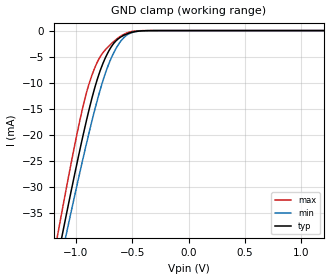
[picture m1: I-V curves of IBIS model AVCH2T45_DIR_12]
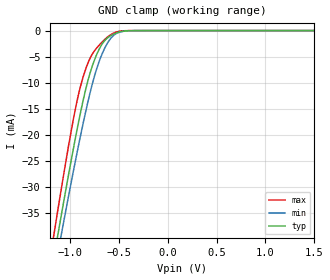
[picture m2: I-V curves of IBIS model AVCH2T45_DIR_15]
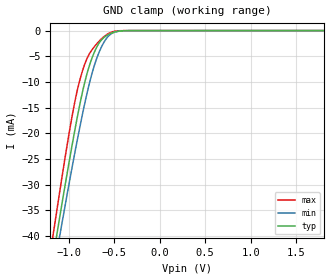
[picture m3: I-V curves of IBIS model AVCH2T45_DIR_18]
| TEXAS INSTRUMENTS INCORPORATED
| Standard Linear and Logic Group
| IBIS Model of SN74AVCH2T45
| DUAL-BIT DUAL-SUPPLY BUS TRANSCEIVER WITH CONFIGURABLE VOLTAGE
| TRANSLATION AND 3-STATE OUTPUTS
| This file contains package information for the following:
|  SOT 8-pin (DCU) package as [Component] AVCH2T45_DCU
|  SOT 8-pin (DCT) package as [Component] AVCH2T45_DCT
|  NanoFree WCSP 8-pin (YZP) package as [Component] AVCH2T45_YZP
| This device can be powered at the following Vccs:
|  1.2 volt Vcc
|  1.5 volt Vcc
|  1.8 volt Vcc
|  2.5 volt Vcc
|  3.3 volt Vcc
| This file provides unique models under the [Model Selector] for each Vcc.
| For operation at a specific Vcc, select the appropriate model after each
| [Model Selector] keyword.
[IBIS Ver]   3.2
[Comment char]  |_char
[File Name]   sn74avch2t45.ibs
[File Rev]   1.2 | x_die
[Date]   December 7, 2005
[Source]   Data created from TI-SPICE simulations at TI-SLL.
[Notes]   The following is an IBIS list for the AVCH2T45.
   Please contact sllibis@ti.com with questions and
   comments concerning SLL IBIS models.
   - FILE REV HISTORY
   - 1.1 Release of IBIS File on 04/29/04
   - 1.2 YZP package added on 12/07/05
   - Power clamp data deleted as there is no power-clamp diode.
   - Due to the fact that the Device is 4.6-V Input/Output
   tolarent, the I/O models has some Non-Monotonic Warnings.
   - Non-monotonic data in ground-clamp due to bus-hold
[Disclaimer] Property of Texas Instruments Incorporated.  Unauthorized
   reproduction and/or distribution is strictly prohibited.
   This product is protected under copyright law.
   Created  2004, (C) Copyright  2004, Texas Instruments
   Incorporated, All Rights Reserved
   UNLESS THERE IS A SIGNED, WRITTEN AGREEMENT TO THE
   CONTRARY, TEXAS INSTRUMENTS (TI) IS PROVIDING THE IBIS
   MODELS  AND WITHOUT ANY WARRANTY, EXPRESSED OR
   IMPLIED.  TI assumes no liability for:
   1) the accuracy of the IBIS models provided to your
   company;
   2) the proper functioning of these IBIS Models in your
   design or for any resulting applications; or
   3) infringement of patents, copyrights or intellectual
   property rights resulting from your use of these IBIS
   models.
   TI provides IBIS Models as a service to our customers.
   You and your company shall not distribute, sell or give
   these models to anyone else without prior written
   permission from TI.
   TI reserves the right to make changes to our products or
   to discontinue any semiconductor product or service
   without notice, and advises our customers to obtain the
   latest version of relevant information to verify, before
   placing orders, that the information being relied on is
   current.
   Please be aware that your receipt and use of the IBIS
   information provided shall serve as acceptance of these
   terms and conditions.  If you do not accept these terms,
   you should return or destroy the IBIS models and any
   other accompanying information immediately.
| Component AVCH2T45_DCU 8-pin SOT
[Component]   AVCH2T45_DCU
[Manufacturer]   Texas Instruments, Inc.
[Package]
|   typ   min   max
R_pkg   2.600e-02   2.300e-02   3.800e-02
L_pkg   1.394e-09   1.066e-09   2.046e-09
C_pkg   2.590e-13   2.150e-13   3.720e-13
[Pin]   signal_name   model_name   R_pin   L_pin   C_pin
1   VCCA   POWER   2.400e-02   1.520e-09   2.710e-13
2   A1   AVCH2T45_IOA   2.300e-02   1.112e-09   2.180e-13
3   A2   AVCH2T45_IOA   2.300e-02   1.070e-09   2.170e-13
4   GND   GND   2.700e-02   2.046e-09   3.720e-13
5   DIR   AVCH2T45_DIR   2.700e-02   1.542e-09   2.730e-13
6   B2   AVCH2T45_IOB   2.300e-02   1.100e-09   2.240e-13
7   B1   AVCH2T45_IOB   2.300e-02   1.066e-09   2.150e-13
8   VCCB   POWER   3.800e-02   1.696e-09   2.800e-13
| Component AVCH2T45_DCT 8-pin SOT
[Component]   AVCH2T45_DCT
[Manufacturer]   Texas Instruments, Inc.
[Package]
|   typ   min   max
R_pkg   2.900e-02   2.800e-02   3.100e-02
L_pkg   1.796e-09   1.666e-09   1.924e-09
C_pkg   2.310e-13   2.210e-13   2.420e-13
[Pin]   signal_name   model_name   R_pin   L_pin   C_pin
1   VCCA   POWER   3.100e-02   1.894e-09   2.230e-13
2   A1   AVCH2T45_IOA   2.800e-02   1.697e-09   2.370e-13
3   A2   AVCH2T45_IOA   3.000e-02   1.722e-09   2.390e-13
4   GND   GND   3.000e-02   1.861e-09   2.210e-13
5   DIR   AVCH2T45_DIR   2.800e-02   1.924e-09   2.280e-13
6   B2   AVCH2T45_IOB   2.900e-02   1.736e-09   2.420e-13
7   B1   AVCH2T45_IOB   2.800e-02   1.666e-09   2.360e-13
8   VCCB   POWER   3.000e-02   1.871e-09   2.220e-13
| Component AVCH2T45_YZP 8-pin NanoFree WCSP
[Component]   AVCH2T45_YZP
[Manufacturer]   Texas Instruments, Inc.
[Package]
|   typ   min   max
R_pkg   0.001   0.001   0.001
L_pkg   0.021nH   0.021nH   0.021nH
C_pkg   0.043pF   0.042pF   0.044pF
[Pin]   signal_name   model_name   R_pin   L_pin   C_pin
1   VCCA   POWER   0.046   2.861nH   0.321pF
2   A1   AVCH2T45_IOA   0.037   2.437nH   0.286pF
3   A2   AVCH2T45_IOA   0.034   2.419nH   0.286pF
4   GND   GND   0.043   2.784nH   0.321pF
5   DIR   AVCH2T45_DIR   0.043   2.784nH   0.321pF
6   B2   AVCH2T45_IOB   0.035   2.420nH   0.286pF
7   B1   AVCH2T45_IOB   0.037   2.437nH   0.286pF
8   VCCB   POWER   0.046   2.860nH   0.321pF
| Model AVCH2T45_DIR
[Model Selector]   AVCH2T45_DIR
AVCH2T45_DIR_12   1.2 volt Vcc
AVCH2T45_DIR_15   1.5 volt Vcc
AVCH2T45_DIR_18   1.8 volt Vcc
AVCH2T45_DIR_25   2.5 volt Vcc
AVCH2T45_DIR_33   3.3 volt Vcc
| Model AVCH2T45_IOA
[Model Selector]   AVCH2T45_IOA
AVCH2T45_IOA_12   1.2 volt Vcc
AVCH2T45_IOA_15   1.5 volt Vcc
AVCH2T45_IOA_18   1.8 volt Vcc
AVCH2T45_IOA_25   2.5 volt Vcc
AVCH2T45_IOA_33   3.3 volt Vcc
| Model AVCH2T45_IOB
[Model Selector]   AVCH2T45_IOB
AVCH2T45_IOB_12   1.2 volt Vcc
AVCH2T45_IOB_15   1.5 volt Vcc
AVCH2T45_IOB_18   1.8 volt Vcc
AVCH2T45_IOB_25   2.5 volt Vcc
AVCH2T45_IOB_33   3.3 volt Vcc
| Models and submodels in the file (15): AVCH2T45_DIR_12 (Input), AVCH2T45_DIR_15 (Input), AVCH2T45_DIR_18 (Input), AVCH2T45_DIR_25 (Input), AVCH2T45_DIR_33 (Input), AVCH2T45_IOA_12 (I/O), AVCH2T45_IOA_15 (I/O), AVCH2T45_IOA_18 (I/O), AVCH2T45_IOA_25 (I/O), AVCH2T45_IOA_33 (I/O), AVCH2T45_IOB_12 (I/O), AVCH2T45_IOB_15 (I/O), AVCH2T45_IOB_18 (I/O), AVCH2T45_IOB_25 (I/O), AVCH2T45_IOB_33 (I/O)
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[Model]   AVCH2T45_DIR_12
Model_type  Input
Vinl=0.385
Vinh=0.845
| variable   typ   min   max
C_comp   2.46pF   2.11pF   2.89pF
[Temperature Range]   40   100   -40
| Ambient temperature   25   85   -40
[Voltage range]   1.2   1.1   1.3
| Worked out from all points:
|   GND clamp passes 1 mA (typ) near -0.58 V on its own axis
[GND Clamp]
| AVCH2T45_DIR_12
|   Voltage   I(typ)   I(min)   I(max)
-4.6V     -459.2mA   -437.9mA   -484.2mA
-1.165V   -43.78mA   -47mA      -39.35mA
-1.115V   -38.35mA   -41.89mA   -33.51mA
-1.09V    -35.67mA   -39.36mA   -30.63mA
-1.065V   -33.02mA   -36.85mA   -27.8mA
-945mV    -20.79mA   -25.16mA   -15.18mA
-840mV    -11.44mA   -15.71mA   -7.485mA
-710mV    -3.942mA   -6.433mA   -2.997mA
-630mV    -1.665mA   -2.889mA   -1.475mA
-555mV    -700.6uA   -964.8uA   -509.7uA
-385mV    -23.61uA   -32.06uA   -5.101uA
1.2V      106.8pA    765.6pA    17.5pA
[Model]   AVCH2T45_DIR_15
Model_type  Input
Vinl=0.49
Vinh=1.04
| variable   typ   min   max
C_comp   2.41pF   2.01pF   2.90pF
[Temperature Range]   40   100   -40
| Ambient temperature   25   85   -40
[Voltage range]   1.5   1.4   1.6
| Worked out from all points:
|   GND clamp passes 1 mA (typ) near -0.58 V on its own axis
[GND Clamp]
| AVCH2T45_DIR_15
|   Voltage   I(typ)   I(min)   I(max)
-4.6V     -459.2mA   -437.9mA   -484.2mA
-1.175V   -44.87mA   -48.03mA   -40.53mA
-1.145V   -41.6mA    -44.95mA   -37mA
-1.12V    -38.89mA   -42.4mA    -34.09mA
-1.095V   -36.21mA   -39.87mA   -31.21mA
-1.07V    -33.55mA   -37.35mA   -28.36mA
-945mV    -20.79mA   -25.16mA   -15.18mA
-840mV    -11.44mA   -15.71mA   -7.485mA
-775mV    -7.058mA   -10.58mA   -4.657mA
-700mV    -3.56mA    -5.9mA     -2.784mA
-545mV    -612.9uA   -811.6uA   -423.5uA
1.5V      118pA      793.8pA    21.88pA
[Model]   AVCH2T45_DIR_18
Model_type  Input
Vinl=0.5775
Vinh=1.2675
| variable   typ   min   max
C_comp   2.36pF   1.92pF   2.90pF
[Temperature Range]   40   100   -40
| Ambient temperature   25   85   -40
[Voltage range]   1.8   1.65   1.95
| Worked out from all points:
|   GND clamp passes 1 mA (typ) near -0.58 V on its own axis
[GND Clamp]
| AVCH2T45_DIR_18
|   Voltage   I(typ)   I(min)   I(max)
-4.6V     -459.2mA   -437.9mA   -484.2mA
-1.185V   -45.97mA   -49.06mA   -41.71mA
-1.155V   -42.69mA   -45.98mA   -38.17mA
-1.13V    -39.97mA   -43.42mA   -35.25mA
-1.105V   -37.28mA   -40.88mA   -32.35mA
-1.08V    -34.61mA   -38.36mA   -29.5mA
-950mV    -21.28mA   -25.63mA   -15.65mA
-840mV    -11.44mA   -15.71mA   -7.485mA
-765mV    -6.504mA   -9.869mA   -4.351mA
-695mV    -3.38mA    -5.644mA   -2.68mA
-540mV    -571.7uA   -743.1uA   -384.3uA
1.8V      129.6pA    822.2pA    26.26pA
